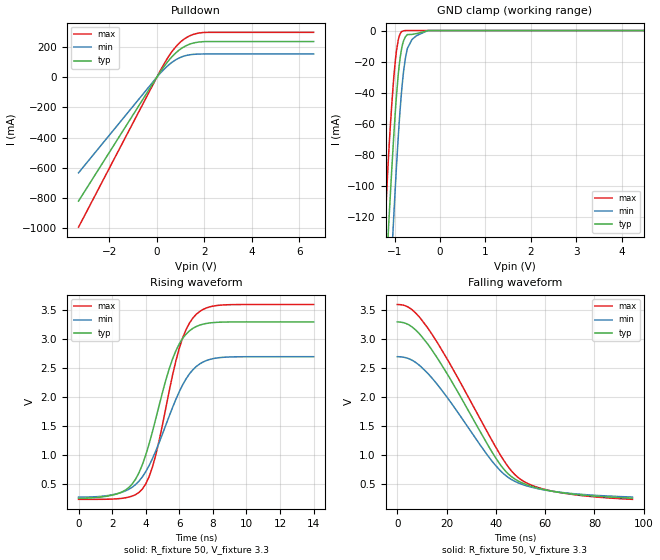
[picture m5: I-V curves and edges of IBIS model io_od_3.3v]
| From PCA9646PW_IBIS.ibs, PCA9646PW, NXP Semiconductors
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[Model]   io_od_3.3v
Model_type I/O_open_drain
Vinl=4.000E-01
Vinh=1.200E+00
Vref=3.300E+00
Rref=2.000E+03
Cref=0.000E+00
Vmeas=1.000E+00
C_comp   1.110E-12   1.080E-12   1.140E-12
[Voltage Range]   3.300E+00   2.700E+00   3.600E+00
[POWER Clamp Reference]   3.300E+00   2.700E+00   3.600E+00
[GND Clamp Reference]   0.000E+00   0.000E+00   0.000E+00
[Pullup Reference]   3.300E+00   2.700E+00   3.600E+00
[Pulldown Reference]   0.000E+00   0.000E+00   0.000E+00
[Temperature Range]   25   85   -40
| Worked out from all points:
|   slope of the pulldown table from 0 to 0.495 V, typ, clamps not added: 4.52 ohm
|   GND clamp passes 1 mA (typ) near -0.39 V on its own axis
|   rising waveform, R_fixture 50, V_fixture 3.3: 20-80 % time 1.8ns typ, 2.11ns min, 1.58ns max; typ from 0.261 V to 3.3 V
|   falling waveform, R_fixture 50, V_fixture 3.3: 20-80 % time 25.3ns typ, 24.8ns min, 26.7ns max; typ from 3.3 V to 0.261 V
[GND Clamp]
-3.3V     -1.424A    -1.555A    -1.323A
-1.2V     -166.7mA   -228mA     -119.2mA
-1.14V    -130.1mA   -189.6mA   -83.9mA
-1.06V    -87.83mA   -143mA     -46.23mA
-1.02V    -68.07mA   -120.1mA   -30.6mA
-920mV    -28.31mA   -68.33mA   -6.065mA
-840mV    -10.77mA   -36.93mA   -505.7uA
-800mV    -6.342mA   -25.61mA   -155.4uA
-720mV    -2.627mA   -11.6mA    0A
-600mV    -2.411mA   -5.305mA   0A
-260mV    0A         0A         0A
6.6V      0A         0A         0A
[Pulldown]
-3.3V     -820.3mA   -633.4mA   -992.9mA
160mV     38.65mA    28.99mA    47.98mA
600mV     129.2mA    93.89mA    161.7mA
840mV     166.3mA    118.7mA    208.3mA
1.04V     190.8mA    133.7mA    238.9mA
1.48V     223.2mA    149.7mA    279.8mA
1.96V     234.6mA    153.1mA    295.2mA
6.6V      235.4mA    153.3mA    296.4mA
[Rising Waveform]
R_fixture = 50
V_fixture = 3.3
V_fixture_min = 2.7
V_fixture_max = 3.6
0s        260.5mV    279.7mV    240.6mV
2.8ns     401.8mV    386.6mV    267.2mV
3.4ns     589.9mV    496.1mV    322mV
4ns       1.004V     716.3mV    505.4mV
4.6ns     1.63V      1.075V     1.006V
5.8ns     2.805V     1.967V     2.632V
6.4ns     3.088V     2.316V     3.166V
7.2ns     3.243V     2.572V     3.477V
8.6ns     3.297V     2.689V     3.592V
14ns      3.3V       2.7V       3.6V
[Falling Waveform]
R_fixture = 50
V_fixture = 3.3
V_fixture_min = 2.7
V_fixture_max = 3.6
0s        3.3V       2.7V       3.6V
5.8ns     3.218V     2.643V     3.515V
12.4ns    2.914V     2.411V     3.192V
21.6ns    2.307V     1.918V     2.558V
39.6ns    975.8mV    838.1mV    1.166V
44.2ns    713.4mV    643.8mV    848.6mV
48.8ns    562.7mV    529.3mV    624.3mV
54.4ns    464.1mV    450.1mV    485.4mV
63ns      379.7mV    379.2mV    380.1mV
95.4ns    260.5mV    279.7mV    240.6mV
[Ramp]
dV/dt_r   1.8237E+00/1.7990E-09   1.4522E+00/2.1080E-09   2.0157E+00/1.5720E-09
dV/dt_f   1.8237E+00/2.5286E-08   1.4522E+00/2.4814E-08   2.0157E+00/2.6733E-08
R_load = 50
